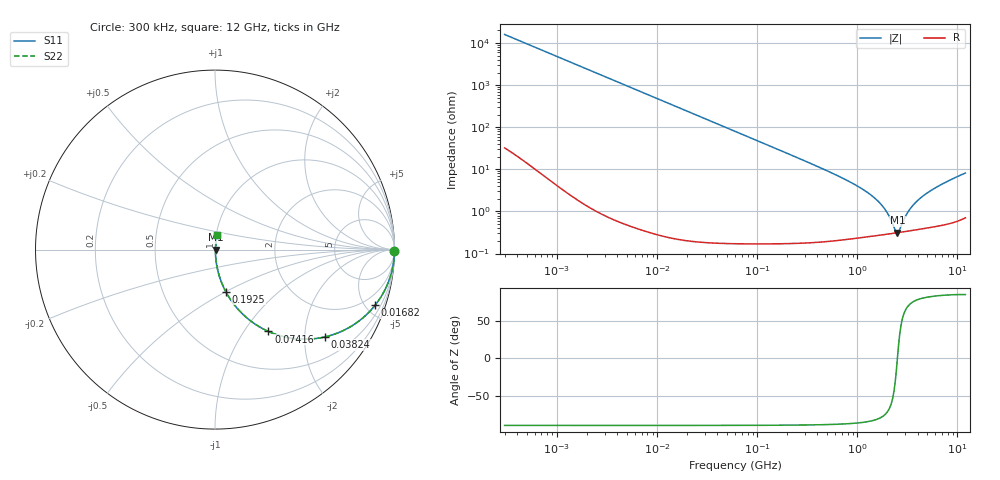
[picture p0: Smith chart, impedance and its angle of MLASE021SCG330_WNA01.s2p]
! MLASE021SCG330_WNA01  S-PARAMETER MODEL  ( Standard Model )
! Model Generated by TAIYO YUDEN Corporation (http://www.ty-top.com)
! Version 2.0
! TAIYO YUDEN Control No. 231201
! Copyright(c) 2022 TAIYO YUDEN CO.,LTD. All Rights Reserved.
! Product Description (link to TY-COMPAS)
! https://ds.yuden.co.jp/TYCOMPAS/or/detail?pn=MLASE021SCG330JWNA01&u=M
! Products Name : Multilayer Ceramic Capacitors
! Characteristics :
!  Capacitance : 33 [pF] , Rated Voltage : 16 [V] , TCC : CG / C0G
!  Case Size : 0.25 x 0.125 / 0.0098 x 0.0049 [mm/inch] , Thickness : 0.125 / 0.0049 [mm/inch]
!  (Conditions: Temperature = 25 [degC] , DC Bias Voltage = 0 [V])
! External Node Assignments :
!  1  o---| |---o  2
! GND o---------o GND
! Frequency Range : 0.3MHz  -  12000MHz  [ 401 STEP ]
# MHZ S RI R 50
! Freq[MHz].  S11 Real  S11 Imag  S21 Real  S21 Imag  S12 Real  S12 Imag  S22 Real  S22 Imag
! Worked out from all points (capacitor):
!   401 points, 300 kHz to 12 GHz, reference 50 ohm
!   read as one part in series: C = 33 pF near 316.3 kHz
!   lowest |Z| = 312 mohm at 2.514 GHz (marker M1)
!   series resonance near 2.513 GHz, so ESL is about 120 pH
!   S11 on the Smith chart (normalised r, x): 300 kHz: open; 16.82 MHz: 1.00, -5.74; 38.24 MHz: 1.00, -2.53; 74.16 MHz: 1.00, -1.30; 192.5 MHz: 1.00, -0.50; 12 GHz: 1.01, +0.16
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0.3  0.9999 -0.00622  5.12e-05 0.00622  5.12e-05 0.00622  0.9999 -0.00622
1.769972  0.9986 -0.0366  0.00136 0.0366  0.00136 0.0366  0.9986 -0.0366
4.716902  0.9905 -0.0967  0.0095 0.0967  0.0095 0.0967  0.9905 -0.0967
10.44266  0.9552 -0.2065  0.0448 0.2065  0.0448 0.2065  0.9552 -0.2065
16.82302  0.8916 -0.3105  0.1084 0.3105  0.1084 0.3105  0.8916 -0.3105
38.24403  0.6144 -0.486  0.3856 0.486  0.3856 0.486  0.6144 -0.486
60  0.3931 -0.4874  0.6069 0.4874  0.6069 0.4874  0.3931 -0.4874
74.16388  0.2979 -0.456  0.7021 0.456  0.7021 0.456  0.2979 -0.456
116.3536  0.1474 -0.3525  0.8526 0.3525  0.8526 0.3525  0.1474 -0.3525
192.4766  0.0599 -0.2339  0.9401 0.2339  0.9401 0.2339  0.0599 -0.2339
353.9943  0.0192 -0.1306  0.9808 0.1306  0.9808 0.1306  0.0192 -0.1306
763.2128  0.00535 -0.0566  0.9946 0.0566  0.9946 0.0566  0.00535 -0.0566
1229.528  0.00333 -0.0293  0.9967 0.0293  0.9967 0.0293  0.00333 -0.0293
1689.663  0.00296 -0.0153  0.997 0.0153  0.997 0.0153  0.00296 -0.0153
2088.533  0.00297 -0.00695  0.997 0.00695  0.997 0.00695  0.00297 -0.00695
2384.334  0.00306 -0.00196  0.9969 0.00196  0.9969 0.00196  0.00306 -0.00196
2514.07  0.00311 1.27e-05  0.9969 -1.27e-05  0.9969 -1.27e-05  0.00311 1.27e-05
2650.866  0.00318 0.00198  0.9968 -0.00198  0.9968 -0.00198  0.00318 0.00198
3276.641  0.00352 0.00991  0.9965 -0.00991  0.9965 -0.00991  0.00352 0.00991
4270.516  0.0042 0.0204  0.9958 -0.0204  0.9958 -0.0204  0.0042 0.0204
6524.734  0.00611 0.04  0.9939 -0.04  0.9939 -0.04  0.00611 0.04
12000  0.0135 0.0799  0.9865 -0.0799  0.9865 -0.0799  0.0135 0.0799
